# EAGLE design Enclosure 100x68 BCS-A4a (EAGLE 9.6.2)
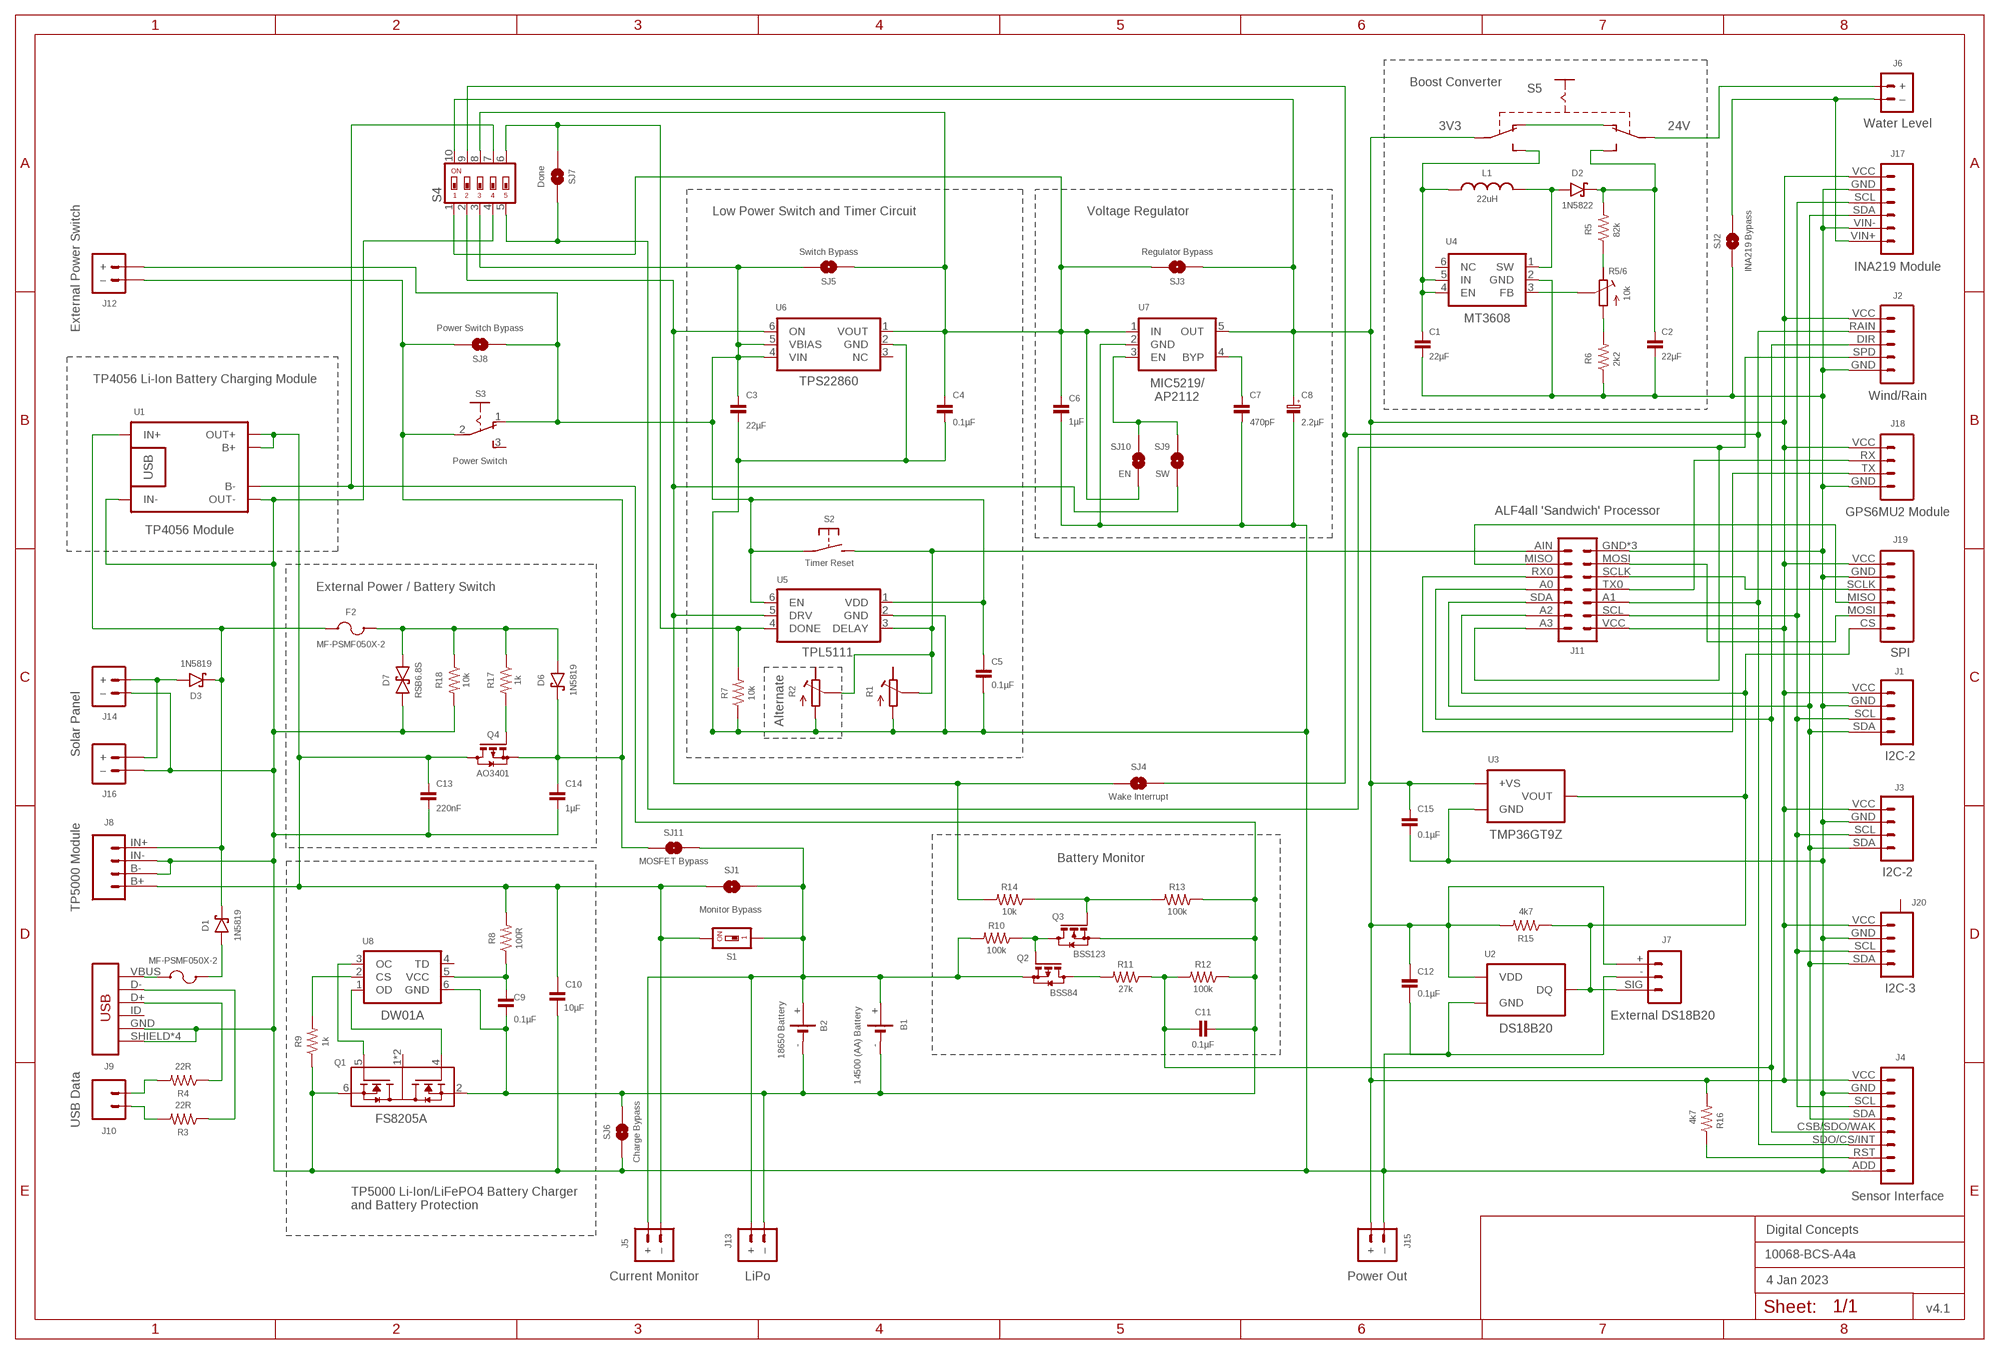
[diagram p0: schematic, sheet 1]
FRAME2 (A3L-LOC): DATE: 4 Jan 2023; OWNER: Digital Concepts; TITLE: 10068-BCS-A4a; VERSION: v4.1

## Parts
B1  14500 (AA) Battery  BATTERY-HOLDER-14500(AA)  [BATTERY-14500]
B2  18650 Battery  BATTERY-HOLDER-18650  [BATTERY-18650]
C1  22µF  CAPACITOR-1206  [C1206]
C2  22µF  CAPACITOR-1206  [C1206]
C3  22µF  CAPACITOR-0805  [C0805]
C4  0.1µF  CAPACITOR-0805  [C0805]
C5  0.1µF  CAPACITOR  [C0805@1]
C6  1µF  CAPACITOR-0805  [C0805]
C7  470pF  CAPACITOR-0805  [C0805]
C8  2.2µF  CAPACITOR-1206-TANTALUM  [C1206-POLARISED]
C9  0.1µF  CAPACITOR-0805  [C0805]
C10  10µF  CAPACITOR-VIA-2  [C0805-VIA-2@1]
C11  0.1µF  CAPACITOR-0805  [C0805]
C12  0.1µF  CAPACITOR-VIA-2  [C0805-VIA-2@1]
C13  220nF  CAPACITOR-0805  [C0805]
C14  1µF  CAPACITOR-0805  [C0805]
C15  0.1µF  CAPACITOR-0805  [C0805]
D1  1N5819  DIODE-SCHOTTKY-1N5819  [SOD-123]
D2  1N5822  DIODE-SCHOTTKY-1N5822  [DIODE_SMB]
D3  1N5819  DIODE-SCHOTTKY-1N5819  [SOD-123]
D6  1N5819  DIODE-SCHOTTKY-1N5819  [SOD-123]
D7  RSB6.8S  DIODE-SCHOTTKY-BIDIRECTIONAL  [VMD2]
F1  MF-PSMF050X-2  [F0805]
F2  MF-PSMF050X-2  [F0805]
J1  I2C-2  JST-PH2.0-4-DUAL-I2C  [JST-PH2.0-4-DUAL-I2C]
J2  Wind/Rain  JST-PH2.0-5-DUAL-WEATHER  [JST-PH2.0-5-DUAL-WEATHER]
J3  I2C-2  HEADER-1X4-I2C  [CONN_04-I2C]
J4  Sensor Interface  HEADER-1X8-SENSOR  [CONN_08-SENSOR]
J5  Current Monitor  JST-PH2.0-2-MALE-HORIZONTALJST-PTH-2  [JST-PH2.0-2-HORIZONTAL]
J6  Water Level  JST-PH2.0-2-MALE-VERTICAL  [JST-PH2.0-2-VERTICAL]
J7  External DS18B20  JST-PH2.0-DS18B20-HORIZONTAL  [JST-PH2.0-DS18B20-HORIZONTAL]
J8  TP5000 Module  HEADER-1X4-TP5000  [CONN_04-TP5000]
J9  USB  USB_MINI-B_SMT  [USB-MINIB]
J10  USB Data  1X2-PIN-HEADER  [CONN_02-GENERIC]
J11  ALF4all 'Sandwich' Processor  ALF4ALL-PROCESSOR-BOARD  [ALF4ALL-PROCESSOR-BOARD]
J12  External Power Switch  JST-PH2.0-2-DUAL-POWERJST-PTH-2  [JST-PH2.0-2-DUAL-POWER]
J13  LiPo  JST-PH2.0-2-MALE-HORIZONTALJST-PTH-2  [JST-PH2.0-2-HORIZONTAL]
J14  Solar Panel  JST-PH2.0-2-VERTICAL  [JST-PH2.0-2-VERTICAL=POWER]
J15  Power Out  JST-SH1.25-2-VERTICAL  [JST-SH1.25-2-VERTICAL]
J16  JST-PH2.0-2-HORIZONTAL-POWERJST-PTH-2  [JST-PH2.0-2-HORIZONTAL-POWER]
J17  INA219 Module  INA219-I2C-MODULE  [CONN_06-INA219]
J18  GPS6MU2 Module  HEADER-1X4-GPS  [CONN_04-GPS]
J19  SPI  JST-PH2.0-6-HORIZONTAL-SPI  [JST-PH2.0-6-HORIZONTAL-SPI]
J20  I2C-3  JST-SH1.0-4-I2C-HORIZONTAL  [JST-SH1.0-4-I2C-HORIZONTAL]
L1  22uH  INDUCTOR-CDRH104R/6D28L5038P  [CDRH104R+6D28]
Q1  FS8205A  MOSFET-DUAL-FS8205A  [FS8205-SOP?]
Q2  BSS84  [SOT23-3@1]
Q3  BSS123  MOSFET-BSS123  [SOT23-3]
Q4  AO3401  MOSFET-AO3401  [SOT-23]
R1  RESISTOR-TRIMM-BAOTER-VERTICAL  [RTRIM3296]
R2  RESISTOR-TRIMM-33  [RTRIM3*3]
R3  22R  RESISTOR-VIA-1  [R0805-VIA-1]
R4  22R  RESISTOR-VIA-1  [R0805-VIA-1]
R5  82k  RESISTORR0805  [R0805]
R5/6  10k  RESISTOR-TRIMM-BAOTER-HORIZONTAL  [RTRIM64P]
R6  2k2  RESISTORR0805  [R0805]
R7  10k  RESISTORR0805  [R0805]
R8  100R  RESISTORR0805  [R0805]
R9  1k  RESISTORR0805  [R0805]
R10  100k  RESISTORR0805  [R0805]
R11  27k  RESISTORR0805  [R0805]
R12  100k  RESISTORR0805  [R0805]
R13  100k  RESISTORR0805  [R0805]
R14  10k  RESISTORR0805  [R0805]
R15  4k7  RESISTORR0805  [R0805]
R16  4k7  RESISTORR0805  [R0805]
R17  1k  RESISTORR0805  [R0805]
R18  10k  RESISTORR0805  [R0805]
S1  Monitor Bypass  SWITCH-DIP-SWS001-VIA-1  [SMD-001-VIA-1]
S2  Timer Reset  SWITCH-MOMENTARY-2-PIN-VIA-1  [SWITCH-2-PAD-VIA-1]
S3  Power Switch  SWITCH-SLIDE-SPDT  [SWITCH-SPDT-PTH]
S4  SWITCH-DIP-SWS005  [SMD-005]
S5  SWITCH-SLIDE-DPDT-PTH-S  [SWITCH-DPDT-PTH]
SJ1  Monitor Bypass  SJ  [SJ]
SJ2  INA219 Bypass  SJ  [SJ]
SJ3  Regulator Bypass  SJ-V-12  [SJ-VIA-12]
SJ4  Wake Interrupt  SJ-V-1  [SJ-VIA-1]
SJ5  Switch Bypass  SJ-V-1  [SJ-VIA-1]
SJ6  Charge Bypass  SJ-V-1  [SJ-VIA-1]
SJ7  Done  SJ-V-1  [SJ-VIA-1]
SJ8  Power Switch Bypass  SJ  [SJ]
SJ9  SW  SJ  [SJ]
SJ10  EN  SJ  [SJ]
SJ11  MOSFET Bypass  SJ  [SJ]
U1  TP4056 Module  BATTERY-CHARGER-LI-PROT  [BATTERY-CHARGER-LI-PROT]
U2  DS18B20  THERMOMETER-DS18B20  [TO-92]
U3  TMP36GT9Z  THERMOMETER-TMP35GT9Z  [TO-92]
U4  MT3608  [SOT-23-6]
U5  TPL5111  TPL5111DDCR  [SOT-23-6]
U6  TPS22860  [SOT-23-6]
U7  MIC5219  [SOT-23-5]
U8  DW01A  [SOT-23-6]

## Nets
GND: C1.2 C2.2 C3.2 C4.1 C5.1 C6.2 C7.2 C8.2(-) C10.2 C10.2@VIA C12.2 C12.2@VIA C13.2 C14.2 C15.2 D7.P$2 J1.GND J2.GND J3.GND J4.ADD J4.GND J7.- J8.B- J8.IN- J9.GND J9.SHIELD J9.SHIELD@2(SHIELD) J9.SHIELD@3(SHIELD) J9.SHIELD@4(SHIELD) J11.GND J11.GND@TL J11.GND@TR J14.-(–) J15.-(–) J16.-(–) J17.GND J17.VIN- J18.GND J19.GND J20.GND Q1.6(S2) R1.1(A) R2.1(A) R6.1 R7.1 R9.1 R18.2 S4.4 SJ2.1 SJ6.1 SJ6.1@V U1.IN- U1.OUT- U2.1(GND) U3.3(GND) U4.2(GND) U5.2(GND) U6.2(GND) U7.2(GND)
N$1: D3.A J14.+ J16.+
N$2: C4.2 C6.1 S4.1 S4.8 SJ3.2 SJ3.2@V SJ5.1 SJ5.1@V SJ10.2 U6.1(VOUT) U7.1(IN)
N$3: R9.2 U8.2(CS)
N$4: J10.2 R4.2
N$5: R7.2 S4.6 SJ7.1 SJ7.1@V U5.4(DONE)
N$6: D2.A L1.1 U4.1(SW)
N$7: C7.1 U7.4(BYP)
N$8: J1.SCL J3.SCL J4.SCL J11.SCL J17.SCL J20.SCL
N$9: J4.RST R16.1
N$10: C11.1 J2.DIR J4.CSB/SDO/WAK J11.A0 R11.1 R12.2
N$11: J1.SDA J3.SDA J4.SDA J11.SDA J17.SDA J20.SDA
N$12: B1.+ B2.+ J5.+ J13.+ Q2.2(S) R10.2 S1.1 S1.1@VIA SJ1.1 SJ11.2
N$13: R5.1 R5/6.3(E)
N$14: J11.TX0 J18.RX
N$15: J6.-(–) J17.VIN+ SJ2.2
N$16: J11.RX0 J18.TX
N$18: Q1.5(G2) U8.3(OC)
N$19: F1.2 J9.VBUS
N$20: Q1.4(G1) U8.1(OD)
N$21: J9.D+ R4.1 R4.1@VIA
N$22: C9.1 R8.1 U8.5(VCC)
N$23: Q2.3(D) R11.2
N$24: J9.D- R3.1 R3.1@VIA
N$25: J11.AIN R1.2(S) R2.2(S) S2.2(S) U5.3(DELAY)
N$26: C3.1 C5.2 J12.+ S2.1(P) S2.1@VIA(P) S3.1(O) S4.3 SJ5.2 SJ8.1 U5.1(VDD) U5.6(EN) U6.4(VIN) U6.5(VBIAS)
N$27: R5/6.1(A) R6.2
N$28: R14.2 S4.2 SJ4.2 SJ9.2 U5.5(DRV) U6.6(ON)
N$29: J2.SPD J11.A3 S4.5 SJ7.2
N$30: J2.RAIN J4.SDO/CS/INT J11.A1 S4.9 SJ4.1 SJ4.1@V
N$31: R5/6.2(S) U4.3(FB)
N$32: C2.1 D2.C R5.2 S5.P$6(S2)
N$33: S5.P$1(O1) S5.P$4(O2)
N$34: C10.1 C13.1 J5.-(–) J8.B+ Q4.3(D) R8.2 S1.2 SJ1.2 U1.B+ U1.OUT+
N$35: Q2.1(G) Q3.3(D) R10.1
N$36: J6.+ S5.P$5(P2)
N$37: Q3.1(G) R13.2 R14.1
N$38: B1.- B2.- C9.2 C11.2 J13.-(–) Q1.2(S1) Q3.2(S) R12.1 R13.1 S4.7 SJ6.2 U1.B- U8.6(GND)
N$39: C1.1 L1.2 S5.P$3(S1) U4.4(EN) U4.5(IN)
N$40: C14.1 D6.C J12.-(–) Q4.2(S) S3.2(P) SJ8.2 SJ11.1
N$41: D1.C D3.C F2.1 J8.IN+ U1.IN+
N$42: J10.1 R3.2
N$43: Q4.1(G) R17.2
N$44: D6.A D7.P$1 F2.2 R17.1 R18.1
N$45: D1.A F1.1
N$46: SJ9.1 SJ10.1 U7.3(EN)
N$47: J11.SCLK J19.SCLK
N$48: J11.MOSI J19.MOSI
N$49: J7.SIG J11.A2 J19.CS R15.1 U2.2(DQ) U3.2(VOUT)
N$50: J11.MISO J19.MISO
VCC: C8.1(+) C12.1 C15.1 J1.VCC J2.VCC J3.VCC J4.VCC J7.+ J11.VCC J15.+ J17.VCC J18.VCC J19.VCC J20.VCC R15.2 R16.2 S4.10 S5.P$2(P1) SJ3.1 SJ3.1@V U2.3(VDD) U3.1(+VS) U7.5(OUT)
Unconnected: J9.ID J20.A@1(A) J20.A@4(A) Q1.1(D12) Q1.8(D12) R1.3(E) R2.3(E) S3.3(S) U4.6(NC) U6.3(NC) U8.4(TD)

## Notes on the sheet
- Boost Converter
- 3V3 | 24V
- Low Power Switch and Timer Circuit | Voltage Regulator
- TP4056 Li-Ion Battery Charging Module
- MIC5219/
  AP2112
- External Power / Battery Switch
- Alternate
- Battery Monitor
- TP5000 Li-Ion/LiFePO4 Battery Charger
  and Battery Protection

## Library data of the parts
B1 = digitalconcepts:BATTERY-HOLDER-14500(AA): 14500 (AA) battery holder
B2 = digitalconcepts:BATTERY-HOLDER-18650: 18650 Battery Holder
C1 C2 = digitalconcepts:CAPACITOR-1206: 1206 Capacitor
C3 C4 C6 C7 C9 C11 C13-C15 = digitalconcepts:CAPACITOR-0805: 0805 Capacitor
C5 = digitalconcepts:CAPACITOR: 0805 Capacitor
C8 = digitalconcepts:CAPACITOR-1206-TANTALUM: Capacitor 1206 Tantalum
C10 C12 = digitalconcepts:CAPACITOR-VIA-2: 0805 Capacitor with via on Pad 2
D1 D3 D6 = digitalconcepts:DIODE-SCHOTTKY-1N5819: 1N5819 Schottky Diode SOD-123
D2 = digitalconcepts:DIODE-SCHOTTKY-1N5822: 1N5822 Schottky Diode SMB
D7 = digitalconcepts:DIODE-SCHOTTKY-BIDIRECTIONAL: Schottky Bidirectional Diode
F1 F2 = digitalconcepts:MF-PSMF050X-2: PTC Resettable Fuse
J1 = digitalconcepts:JST-PH2.0-4-DUAL-I2C: PH2.0 4P I2C Dual Connector
J2 = digitalconcepts:JST-PH2.0-5-DUAL-WEATHER: PH2.0 5P Vertical Connector
J3 = digitalconcepts:HEADER-1X4-I2C: I2C Interface [Pin 1 Vcc] 4-Pin Header
J4 = digitalconcepts:HEADER-1X8-SENSOR: IoT Sensors 1x8 Pin Header for 'Sandwich' IoT Sensors
J5 J13 = digitalconcepts:JST-PH2.0-2-MALE-HORIZONTAL: PH2.0 2P Right Angle PCB Connector; PROD_ID: CONN-09863; SKU: PRT-09914
J6 = digitalconcepts:JST-PH2.0-2-MALE-VERTICAL: PH2.0 2P PCB Connector
J7 = digitalconcepts:JST-PH2.0-DS18B20-HORIZONTAL: DS18B20 PH2.0 Right Angle PCB Connector
J8 = digitalconcepts:HEADER-1X4-TP5000: TP5000 Module 4-Pin Header
J9 = digitalconcepts:USB_MINI-B: USB Mini-B Connector Breaks out 5 pins, and includes shield pins if needed.
J10 = digitalconcepts:1X2-PIN-HEADER: Single Row 2-Pin Header
J11 = digitalconcepts:ALF4ALL-PROCESSOR-BOARD: ALF4all 'Sandwixh' Processor 2x7 Pin Header and earthed 1x1 locator pins for ALF4all 'Sandwich' Processor/RFM95W PCBs
J12 = digitalconcepts:JST-PH2.0-2-DUAL-POWER: JST PH2.0 2P PTH Dual-Side Connector (Power); PROD_ID: CONN-09863; SKU: PRT-09914
J14 = digitalconcepts:JST-PH2.0-2-VERTICAL: PH2.0 2P PCB Connector
J15 = digitalconcepts:JST-SH1.25-2-VERTICAL: SH1.25 Male PCB Connector
J16 = digitalconcepts:JST-PH2.0-2-HORIZONTAL-POWER: PH2.0 2P Right Angle PCB Connector; PROD_ID: CONN-09863; SKU: PRT-09914
J17 = digitalconcepts:INA219-I2C-MODULE: INA219 I2C Module
J18 = digitalconcepts:HEADER-1X4-GPS: NEO GPS 4-Pin Header
J19 = digitalconcepts:JST-PH2.0-6-HORIZONTAL-SPI: PH2.0 6P Horizontal Connector—SPI
J20 = digitalconcepts:JST-SH1.0-4-I2C-HORIZONTAL: JST SH1.0 SMD 4P I2C horizontal connector
L1 = digitalconcepts:INDUCTOR-CDRH104R/6D28: Inductor; SPICEPREFIX: L
Q1 = digitalconcepts:MOSFET-DUAL-FS8205A: Dual MOSFET; AVAILABILITY: Unavailable; MF: Fortune Semiconductor; MP: FS8205A; PACKAGE: Package; PRICE: None
Q2 = digitalconcepts:BSS84: P-CHANNEL MOS FET
Q3 = digitalconcepts:MOSFET-BSS123: N-CHANNEL MOS FET
Q4 = digitalconcepts:MOSFET-AO3401: AO3401 P-Channel MOSFET
R1 = digitalconcepts:RESISTOR-TRIMM-BAOTER-VERTICAL: Trimm Resistor - Vertical BAOTER
R2 = digitalconcepts:RESISTOR-TRIMM-3*3: Trimm Resistor - 3*3 SMD
R3 R4 = digitalconcepts:RESISTOR-VIA-1: Resistor with via on Pad 1
R5-R18 = digitalconcepts:RESISTOR: Resistor; SPICEPREFIX: R
R5/6 = digitalconcepts:RESISTOR-TRIMM-BAOTER-HORIZONTAL: Trimm Resistor - Horizontal BAOTER
S1 = digitalconcepts:SWITCH-DIP-SWS001-VIA-1: SMD Dip Switch 1 pol.
S2 = digitalconcepts:SWITCH-MOMENTARY-2-PIN-VIA-1: 2 Pin Momentary Switch
S3 = digitalconcepts:SWITCH-SLIDE-SPDT: Mini Sliding Switch SPDT
S4 = digitalconcepts:SWITCH-DIP-SWS005: SMD Dip Switch 5 pol.
S5 = digitalconcepts:SWITCH-SLIDE-DPDT-PTH-S: Switch DPDT PTH-S
SJ1 SJ2 SJ8-SJ11 = digitalconcepts:SJ: Solder Jumper
SJ3 = digitalconcepts:SJ-V-12: Solder Jumper with Pad Vias
SJ4-SJ7 = digitalconcepts:SJ-V-1: Solder Jumper with single Pad Via
U1 = digitalconcepts:BATTERY-CHARGER-LI-PROT: TP4056 Li Battery Charger module with PCB (rather than module) footprint
U2 = digitalconcepts:THERMOMETER-DS18B20: Digital Thermometer -55C-125C TO92-3; AVAILABILITY: Bad; DESCRIPTION: Temperature Sensor Digital, Local -55°C ~ 125°C 12 b 8-uMAX; MF: Maxim Integrated; MP: DS18B20; PACKAGE: TO-92 Maxim Integrated; PRICE: None
U3 = digitalconcepts:THERMOMETER-TMP35GT9Z: Temperature Sensor; AVAILABILITY: Warning; DESCRIPTION: Temperature Sensor Analog, Local 10°C ~ 125°C 10mV/°C TO-92-3; MF: Analog Devices; MOUSER-PURCHASE-URL: https://snapeda.com/shop?store=Mouser&id=409845; MP: TMP35GT9Z; PACKAGE: TO-92-3 Analog Devices; PRICE: None
U4 = digitalconcepts:MT3608: MT3608 DC-DC Step-Up Voltage Converter
U5 = digitalconcepts:TPL5111DDCR: TPL5111 Nano-Power System Timer
U6 = digitalconcepts:TPS22860: Texas Instruments TPS22860 Ultra-Low Leakage Load Switch
U7 = digitalconcepts:MIC5219: Microchip LDO Linear Voltage Regulator; OC_FARNELL: unknown; OC_NEWARK: unknown
U8 = digitalconcepts:DW01A: Battery Protection IC; AVAILABILITY: Unavailable; DESCRIPTION: One Cell Lithium-ion/Polymer Battery Protection IC; MF: Fortune Semiconductor; MP: DW01A; PACKAGE: SOT-23-6 Fortune Semiconductor; PRICE: None

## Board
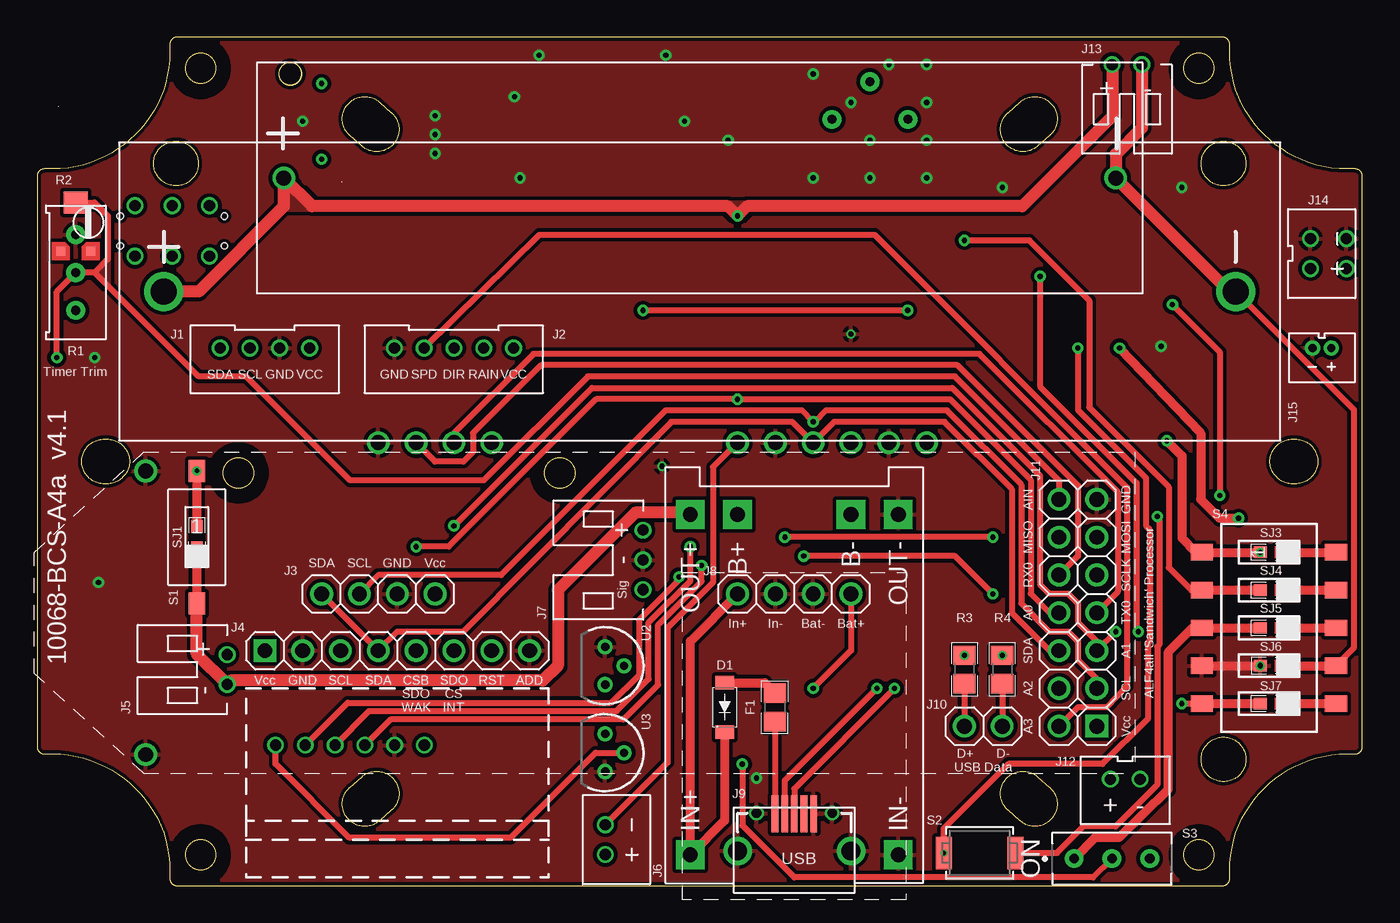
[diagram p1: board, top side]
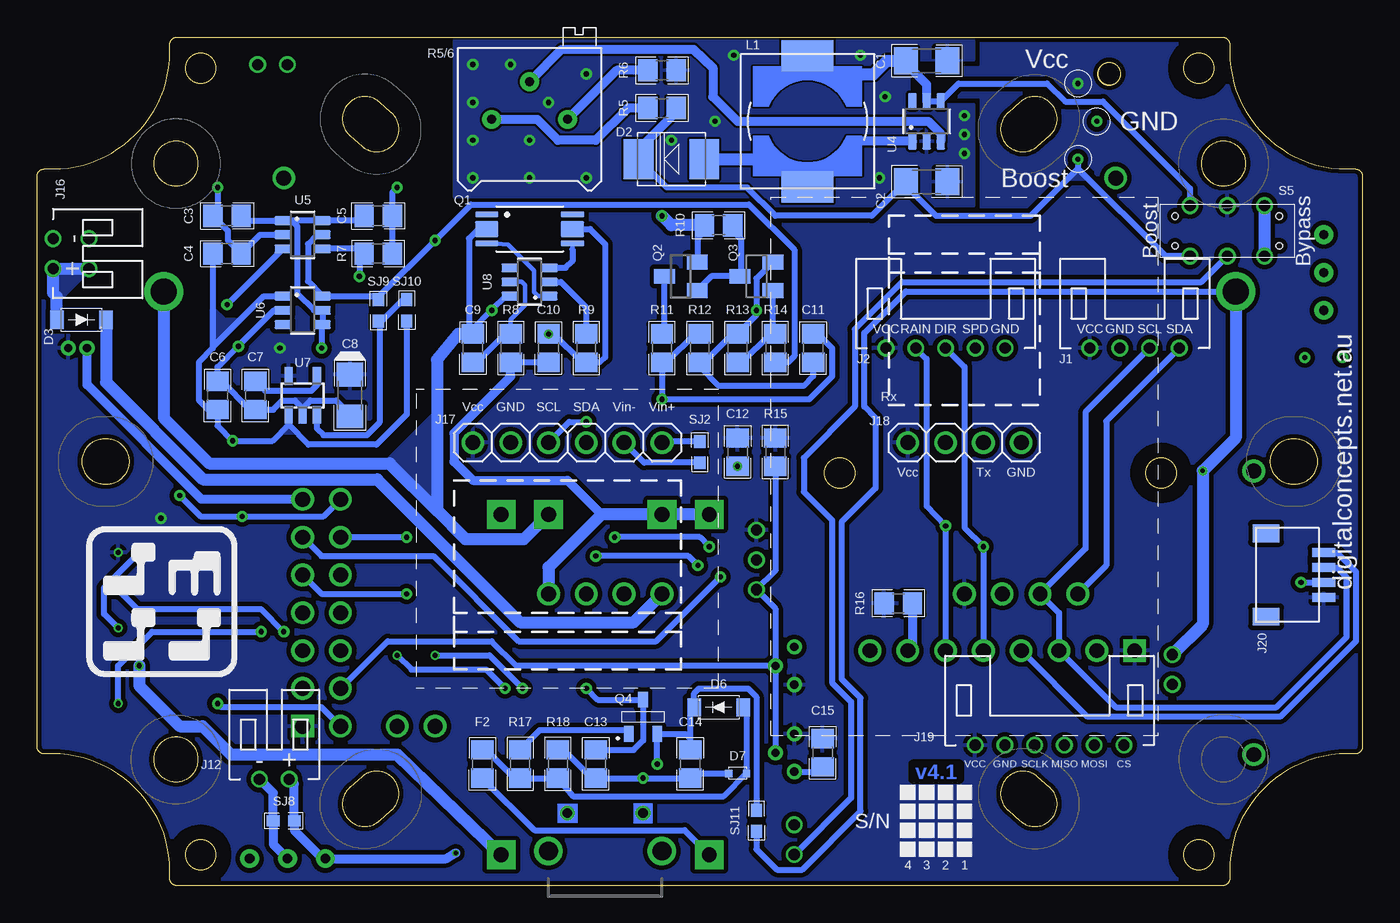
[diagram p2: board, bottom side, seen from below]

Size 89 x 57 mm. Coordinates in mm from the lower left corner, seen from the top.
Outline: 1146 segments
Outline: circle at 17,54.54 radius 0.76
Outline: circle at 10.97,54.91 radius 1.02
Outline: circle at 10.97,2.08 radius 1.02
Outline: circle at 13.51,27.73 radius 1.02
Outline: circle at 35.1,27.73 radius 1.02
Outline: circle at 78.03,2.08 radius 1.02
Outline: circle at 78.03,54.91 radius 1.02
Copper layers (1*16): Top 0.035mm / dielectric 1.5mm / Bottom 0.035mm
Design rules "default *": minimum track width 6mil, minimum drill 0.3mm, track to track 6mil, track to pad 6mil, pad to pad 6mil, via to via 6mil, smd to smd 6mil, copper to edge 6mil, drill to drill 6mil, minimum pad ring 1mil, minimum via ring 8mil, stop-mask expansion 4mil, vias tented up to drill 0mil, thermal gap 10mil

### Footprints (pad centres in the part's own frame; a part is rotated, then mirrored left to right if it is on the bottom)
BATTERY-14500 = drill 1: + -27.94,0; - 27.94,0
BATTERY-18650 = drill 1.75: + -36,0; - 36,0
C1206 = smd 1.6 x 1.8: 1 -1.4,0; 2 1.4,0
C0805 = smd 1.3 x 1.5: 1 -0.95,0; 2 0.95,0
C0805@1 = smd 1.3 x 1.5: 1 -0.95,0; 2 0.95,0
C1206-POLARISED = smd 1.6 x 1.8: 1 -1.4,0; 2 1.4,0
C0805-VIA-2@1 = smd 1.3 x 1.5: 1 -0.95,0; 2 0.95,0 | drill 0.35 pad 0.61: 2@VIA 0.95,0
SOD-123 = smd 0.91 x 1.22: A -1.65,0; C 1.65,0
DIODE_SMB = smd 2 x 2.7: A 2.2,0; C -2.2,0
VMD2 = smd 0.5 x 0.5: P$1 -0.6,0; P$2 0.6,0
F0805 = smd 1.3 x 1.5: 1 -0.95,0; 2 0.95,0
JST-PH2.0-4-DUAL-I2C = drill 0.75: GND -1,0; SCL 1,0; SDA 3,0; VCC -3,0
JST-PH2.0-5-DUAL-WEATHER = drill 0.75: DIR 0,0; GND 4,0; RAIN -2,0; SPD 2,0; VCC -4,0
CONN_04-I2C = drill 1 pad 1.524: GND 2.54,0; SCL 5.08,0; SDA 7.62,0; VCC 0,0
CONN_08-SENSOR = drill 1 pad 1.524: ADD 17.78,0; CSB/SDO/WAK 10.16,0; GND 2.54,0; RST 15.24,0; SCL 5.08,0; SDA 7.62,0; SDO/CS/INT 12.7,0 | drill 1 pad 1.524 square: VCC 0,0
JST-PH2.0-2-HORIZONTAL = drill 0.75: + 1,0; - -1,0
JST-PH2.0-2-VERTICAL = drill 0.75: + -1,0; - 1,0
JST-PH2.0-DS18B20-HORIZONTAL = drill 0.75: + 2,0; - 0,0; SIG -2,0
CONN_04-TP5000 = drill 1 pad 1.524: B+ 0,0; B- 2.54,0; IN+ 7.62,0; IN- 5.08,0
USB-MINIB = smd 2.5 x 0.45: D+ 2.5,0; D- 2.5,0.65; GND 2.5,-1.3; ID 2.5,-0.65; VBUS 2.5,1.3 | drill 1.27: SHIELD 0,3.81; SHIELD@2 0,-3.81 | drill 0.65 pad 0.762: SHIELD@3 2.54,2.54; SHIELD@4 2.54,-2.54
CONN_02-GENERIC = drill 1 pad 1.524: 1 0,0; 2 2.54,0
ALF4ALL-PROCESSOR-BOARD = drill 1 pad 1.524: A0 7.62,2.54; A1 5.08,0; A2 2.54,2.54; A3 0,2.54; AIN 15.24,2.54; GND 15.24,0; GND@TL -1.905,63.881; GND@TR 17.145,63.881; MISO 12.7,2.54; MOSI 12.7,0; RX0 10.16,2.54; SCL 2.54,0; SCLK 10.16,0; SDA 5.08,2.54; TX0 7.62,0 | drill 1 pad 1.524 square: VCC 0,0
JST-PH2.0-2-DUAL-POWER = drill 0.75: + 1,0; - -1,0
JST-PH2.0-2-VERTICAL=POWER = drill 0.75: + -1,0; - 1,0
JST-SH1.25-2-VERTICAL = drill 0.55 pad 1.016: + 0.625,0; - -0.625,0
JST-PH2.0-2-HORIZONTAL-POWER = drill 0.75: + 1,0; - -1,0
CONN_06-INA219 = drill 1 pad 1.524: GND 2.54,0; SCL 5.08,0; SDA 7.62,0; VCC 0,0; VIN+ 12.7,0; VIN- 10.16,0
CONN_04-GPS = drill 1 pad 1.524: GND 0,0; RX 5.08,0; TX 2.54,0; VCC 7.62,0
JST-PH2.0-6-HORIZONTAL-SPI = drill 0.75: CS 5,0; GND -3,0; MISO 1,0; MOSI 3,0; SCLK -1,0; VCC -5,0
JST-SH1.0-4-I2C-HORIZONTAL = smd 1.2 x 1.8: A@1 -2.8,-3.875; A@4 2.8,-3.875 | smd 0.6 x 1.55: GND 0.5,0; SCL -0.5,0; SDA -1.5,0; VCC 1.5,0
CDRH104R+6D28 = smd 2.1 x 3.5: 1 -4.4,0; 2 4.4,0
FS8205-SOP? = smd 1.56 x 0.4: 1 -2.88,0.975; 4 -2.88,-0.975; 5 2.88,-0.975; 8 2.88,0.975 | smd 1.56 x 1.05: 2 -2.88,0; 6 2.88,0
SOT23-3@1 = smd 1 x 1.4: 1 -0.95,-1.1; 2 0.95,-1.1; 3 0,1.1
SOT23-3 = smd 1 x 1.4: 1 -0.95,-1.1; 2 0.95,-1.1; 3 0,1.1
SOT-23 = smd 0.65 x 1.05: 1 -0.95,-1.15; 2 0.95,-1.15; 3 0,1.15
RTRIM3296 = drill 0.61 pad 1.27: 1 0,-2.54; 2 0,0; 3 0,2.54
RTRIM3*3 = smd 0.6 x 0.6: 1 -1,-1.6; 3 1,-1.6 | smd 1.6 x 1.5: 2 0,1.65
R0805-VIA-1 = smd 1.3 x 1.5: 1 -0.95,0; 2 0.95,0 | drill 0.35 pad 0.61: 1@VIA -0.95,0
R0805 = smd 1.3 x 1.5: 1 -0.95,0; 2 0.95,0
RTRIM64P = drill 0.61 pad 1.27: 1 0,-2.54; 2 2.54,0; 3 0,2.54
SMD-001-VIA-1 = smd 1.1 x 1.5: 1 0,-4.45; 2 0,4.45 | drill 0.3 pad 0.61: 1@VIA 0,-4.45
SWITCH-2-PAD-VIA-1 = smd 1.067 x 2.184: 1 -2.4,0; 2 2.4,0 | drill 0.3: 1@VIA -2.4,0
SWITCH-SPDT-PTH = drill 0.65 pad 1.27: 1 -2.54,0; 2 0,0; 3 2.54,0
SMD-005 = smd 1.1 x 1.5: 1 -5.08,-4.5; 2 -2.54,-4.5; 3 0,-4.5; 4 2.54,-4.5; 5 5.08,-4.5; 6 5.08,4.5; 7 2.54,4.5; 8 0,4.5; 9 -2.54,4.5; 10 -5.08,4.5
SWITCH-DPDT-PTH = drill 0.75: P$1 -1.7,2.5; P$2 -1.7,0; P$3 -1.7,-2.5; P$4 1.7,2.5; P$5 1.7,0; P$6 1.7,-2.5 | hole 0.42: 1,3.5; -1,3.5; 1,-3.5; -1,-3.5
SJ = smd 0.864 x 0.762: 1 -0.711,0; 2 0.711,0
SJ-VIA-12 = smd 0.864 x 0.762: 1 -0.711,0; 2 0.711,0 | drill 0.35 pad 0.61: 1@V -0.711,0; 2@V 0.711,0
SJ-VIA-1 = smd 0.864 x 0.762: 1 -0.711,0; 2 0.711,0 | drill 0.35 pad 0.61: 1@V -0.711,0
BATTERY-CHARGER-LI-PROT = drill 1 pad 1.93 square: B+ 10.795,3.81; B- 10.795,-3.81; IN+ -12.065,6.985; IN- -12.065,-6.985; OUT+ 10.795,6.985; OUT- 10.795,-6.985
TO-92 = drill 0.55 pad 1.016: 1 -1.27,0; 2 0,1.27; 3 1.27,0
SOT-23-6 = smd 1.1 x 0.6: 1 -1.35,0.95; 2 -1.35,0; 3 -1.35,-0.95; 4 1.35,-0.95; 5 1.35,0; 6 1.35,0.95
SOT-23-5 = smd 0.55 x 1.2: 1 -0.95,-1.3; 2 0,-1.3; 3 0.95,-1.3; 4 0.95,1.3; 5 -0.95,1.3

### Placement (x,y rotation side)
B1  44.5,47.54 0 top
B2  44.5,39.92 0 top
C1  29.26,55.42 0 bottom
C2  29.26,47.29 0 bottom
C3  76.25,45 180 bottom
C4  76.25,42.46 180 bottom
C5  66.09,45 180 bottom
C6  76.88,32.94 90 bottom
C7  74.34,32.94 270 bottom
C8  67.99,32.94 270 bottom
C9  59.74,36.11 90 bottom
C10  54.66,36.11 90 bottom
C11  36.88,36.11 270 bottom
C12  41.96,29.13 270 bottom
C13  51.48,8.17 270 bottom
C14  45.13,8.17 270 bottom
C15  36.24,8.93 270 bottom
D1  46.18,11.98 270 top
D2  46.4,48.81 0 bottom
D3  86.03,38.02 0 bottom
D6  43.23,11.98 180 bottom
D7  41.96,7.54 180 bottom
F1  49.55,11.98 270 top
F2  59.1,8.17 90 bottom
J1  15.29,36.11 0 bottom
J2  27.99,36.11 0 bottom
J3  26.72,19.6 180 top
J4  15.29,15.79 0 top
J5  12.75,14.52 90 top
J6  38.15,3.09 90 top
J7  40.69,21.89 90 top
J8  54.66,19.6 180 top
J9  50.85,2.33 90 top
J10  62.28,10.71 0 top
J11  71.17,10.71 90 top
J12  73.07,7.16 0 bottom
J13  73.2,55.16 180 top
J14  85.52,42.46 90 top
J15  86.28,36.11 0 top
J16  87.93,42.46 270 bottom
J17  59.74,29.76 0 bottom
J18  22.91,29.76 180 bottom
J19  21,9.44 0 bottom
J20  2.59,20.87 270 bottom
L1  37.26,51.35 90 bottom
Q1  55.93,44.11 0 bottom
Q2  45.77,40.94 90 bottom
Q3  40.69,40.94 90 bottom
Q4  48.31,11.35 0 bottom
R1  2.59,41.19 180 top
R2  2.59,44.24 0 top
R3  62.28,14.52 270 top
R4  64.82,14.52 270 top
R5  47.04,52.24 0 bottom
R5/6  55.93,51.48 90 bottom
R6  47.04,54.78 180 bottom
R7  66.09,42.46 180 bottom
R8  57.2,36.11 270 bottom
R9  52.12,36.11 90 bottom
R10  43.23,44.37 180 bottom
R11  47.04,36.11 90 bottom
R12  44.5,36.11 90 bottom
R13  41.96,36.11 270 bottom
R14  39.42,36.11 270 bottom
R15  39.42,29.13 90 bottom
R16  31.16,18.97 180 bottom
R17  56.56,8.17 90 bottom
R18  54.02,8.17 90 bottom
S1  10.72,23.41 180 top
S2  63.3,2.2 0 top
S3  72.19,1.82 0 top
S4  82.73,17.32 270 top
S5  9.07,43.99 270 bottom
SJ1  10.72,23.41 270 top
SJ2  44.5,29.13 90 bottom
SJ3  82.85,22.4 180 top
SJ4  82.85,19.86 180 top
SJ5  82.85,17.32 180 top
SJ6  82.85,14.78 0 top
SJ7  82.85,12.24 180 top
SJ8  72.44,4.36 180 bottom
SJ9  66.09,38.65 90 bottom
SJ10  64.18,38.65 270 bottom
SJ11  40.69,4.36 270 bottom
U1  50.85,14.14 90 top
U2  38.15,14.78 270 top
U3  38.15,8.93 270 top
U4  29.26,51.35 90 bottom
U5  71.17,43.73 0 bottom
U6  71.17,38.65 0 bottom
U7  71.17,32.94 0 bottom
U8  55.93,40.56 180 bottom

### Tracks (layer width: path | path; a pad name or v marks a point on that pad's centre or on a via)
$X0
  cutout Bottom: 10.97,56.94 arc180 10.97,52.88 arc180
$X1
  cutout Bottom: 78.03,56.94 arc180 78.03,52.88 arc180
$X2
  cutout Bottom: 78.03,4.11 arc180 78.03,0.04 arc180
$X3
  cutout Bottom: 10.97,4.11 arc180 10.97,0.04 arc180
$X4
  cutout Top: 10.97,56.94 arc180 10.97,52.88 arc180
$X5
  cutout Top: 78.03,56.94 arc180 78.03,52.88 arc180
$X6
  cutout Top: 78.03,4.11 arc180 78.03,0.04 arc180
$X7
  cutout Top: 10.97,4.11 arc180 10.97,0.04 arc180
$X8
  cutout Bottom: 13.51,29.76 arc180 13.51,25.7 arc180
$X9
  cutout Top: 35.1,29.76 arc180 35.1,25.7 arc180
$X10
  cutout Top: 13.51,29.76 arc180 13.51,25.7 arc180
$X11
  cutout Bottom: 35.1,29.76 arc180 35.1,25.7 arc180
GND  (via drill 0.35)
  Top 0.61: S4.4 SJ6.1@V
  Bottom 0.406: D7.P$2 44.82,7.54 C14.2 v48.31,7.22 C13.2 51.74,7.22 53.64,9.12 R18.2 | C10.2@VIA 54.3,37.06 52.4,35.16 R9.1 51.24,35.16 50.85,35.5 50.85,43.1 51.87,44.11 Q1.6 | R7.1 C5.1 65.14,46.59 v64.82,46.91 | U5.2 74.03,43.73 C4.1 76.19,43.36 76.19,43.99 C3.2 76.88,45.32 v76.88,46.91 | U3.3 36.56,7.66 C15.2 | v4.11,20.37 J20.GND | C8.2 67.99,31.67 68.92,32.59 70.64,32.59 71.17,32.07 | U6.2 73.07,38.65 v75.49,36.24 76.88,34.84 C6.2 76.63,33.89 74.73,31.99 C7.2 73.15,31.99 72.54,32.59 71.7,32.59 71.17,32.07 | U7.2 71.17,32.07 | SJ2.1 48.23,28.42 J17.VIN-
  Bottom 0.61: J15.- 85.66,33.66 77.95,25.95 J11.GND
  Bottom 0.813: U1.IN- 64.82,8.81 76,8.81 77.9,10.71 79.42,10.71 82.14,13.43 SJ6.1@V
  other vias: 26.72,51.73 26.72,50.46 26.72,49.19 46.4,50.08 32.05,53 52.12,47.54 55.93,47.54 59.74,55.16 59.74,52.62 52.12,54.53 55.93,50.08 59.74,47.54 59.74,50.08 42.21,55.8 43.48,51.35 32.43,47.54 17.83,51.35 3.86,35.48 33.7,55.8 57.2,55.16 54.66,52.62
  pour Top (isolate 0.254, rank 5): -2.92,59.5 -2.92,-2.56 91.86,-2.56 91.86,59.5
  pour Bottom (rank 2): 61.01,57.07 26.08,57.07 26.08,55.44 30.4,55.44 30.4,52.5 26.08,52.5 26.08,45.64 39.42,45.64 40.05,46.27 61.01,46.27
  pour Bottom (no thermals): 71.17,32.07 70.64,32.59 71.7,32.59
N$1
  Bottom 0.813: D3.A 87.68,39.56 87.93,39.81 J16.+ J14.+
  pour Bottom (no thermals): 87.68,41.46 85.77,41.46 87.68,39.56
N$2  (via drill 0.35)
  Top 0.61: v75.87,29.89 76.88,28.87 76.88,23.35 77.83,22.4 S4.1 SJ3.2@V | SJ5.1@V S4.8
  Bottom 0.406: 72.12,30.97 73.2,29.89 v75.87,29.89 76.88,30.91 C6.1 77.52,31.99 78.15,32.62 78.15,35.16 77.2,36.11 77.2,36.18 | SJ3.2@V 84.5,20.03 84.5,18.26 SJ5.1@V | C4.2 77.2,36.18 | 72.12,30.97 70.79,29.64 66.22,29.64 64.18,31.67 SJ10.2 | 72.12,30.97 U7.1 | 77.2,36.18 73.78,39.6 U6.1
  pour Bottom (no thermals): 77.2,38.72 76.46,37.97 75.4,37.97 77.2,36.18
  pour Bottom (no thermals): 72.56,30.52 71.68,30.52 72.12,30.97
N$3
  Bottom 0.406: U8.2 53.82,40.56 52.14,38.88 52.14,37.09 R9.2
N$4
  Top 0.406: R4.2 J10.2
N$5  (via drill 0.35)
  Top 0.406: v73.96,17.06 73.84,17.19 73.84,27.07 67.36,33.55 v67.36,40.94
  Top 0.61: SJ7.1@V S4.6
  Bottom 0.406: U5.4 66.72,42.78 R7.2 67.36,42.14 v67.36,40.94 | SJ7.1@V 83.56,14.78 81.28,17.06 v73.96,17.06
N$6
  Bottom 0.61: L1.1 36.31,48.3 35.66,48.3 33.96,50 U4.1
  Bottom 0.813: D2.A 39.9,48.81 39.42,48.3 38.21,48.3 L1.1
N$7
  Bottom 0.406: U7.4 70.22,33.6 70.57,33.25 73.71,33.25 C7.1
N$8  (via drill 0.35)
  Top 0.406: J11.SCL 71.17,13.89 69.9,15.16 69.9,16.43 69.26,17.06 67.99,17.06 66.09,18.97 66.09,26.94 61.11,31.92 52.99,31.92 52.23,31.16 v52.12,31.16 51.36,31.92 42.21,31.92 31.16,20.87 22.91,20.87 J3.SCL
  Bottom 0.406: v52.12,31.16 53.26,31.16 J17.SCL | J1.SCL 18.59,31.81 18.59,22.65 J3.SCL 20.37,18.33 J4.SCL 16.56,11.98 5.76,11.98 1.07,16.68 1.07,20.74 1.7,21.37 J20.SCL
N$9
  Bottom 0.61: J4.RST 30.21,16.11 R16.1
N$10  (via drill 0.35)
  Top 0.406: v25.45,22.78 27.63,22.78 37.54,32.68 v47.04,32.68 61.29,32.68 66.72,27.25 66.72,19.6 67.99,18.33 J11.A0
  Bottom 0.406: J4.CSB/SDO/WAK v25.45,22.78 26.72,24.05 26.72,34.84 J2.DIR | R12.2 44.83,37.06 46.73,35.16 R11.1 v47.04,32.68 37.13,32.68 35.61,34.21 35.61,36.11 36.24,36.75 36.56,36.75 C11.1
N$11
  Top 0.406: J11.SDA 67.99,15.79 65.45,18.33 65.45,26.64 60.93,31.16 53.52,31.16 J17.SDA 50.72,31.16 42.59,31.16 28.6,17.06 24.18,17.06 J4.SDA J3.SDA
  Bottom 0.406: J4.SDA 18.46,11.35 5.51,11.35 0.43,16.43 0.43,21.1 1.7,22.37 J20.SDA | J3.SDA 17.19,21.51 17.19,31.21 J1.SDA
N$12  (via drill 0.35)
  Top 0.61: S1.1@VIA SJ1.1
  Top 0.813: J13.+ 72.2,51.68 66.16,45.64 47.67,45.64 v47.04,45 46.4,45.64 18.46,45.64 B1.+ 16.56,45.64 10.84,39.92 B2.+
  Bottom 0.406: R10.2 44.18,43.96 44.64,43.5 44.64,41.92 Q2.2 | SJ11.2 40.69,2.46 39.32,1.09 37.62,1.09 33.7,5 33.7,12.62 34.97,13.89 34.97,24.43 32.69,26.71 32.69,31.41 33.45,32.18 33.45,37.13 30.66,39.92 B2.+
  Bottom 0.813: J5.+ 10.72,17.55 S1.1@VIA 8.5,30.08 B2.+ | v47.04,45 46.4,44.37 R10.2
  pour Top: 16.56,47.54 18.46,45.64 16.56,45.64
  pour Top (no thermals): 47.04,45 46.4,45.64 47.67,45.64
N$13
  Bottom 0.61: R5.1 49.33,52.24 51.48,50.08 54.02,50.08 55.42,51.48 R5/6.3
N$14
  Top 0.406: J11.TX0 72.57,19.73 72.57,26.46 63.3,35.73 33.32,35.73 27.99,30.4 J18.RX
N$15
  Top 0.406: J6.- 42.34,8.28 42.34,17.32 45.39,20.36 45.39,28.11 J17.VIN+
  Bottom 0.406: SJ2.2 46.96,29.84 J17.VIN+
N$16
  Top 0.406: J11.RX0 69.9,22.14 69.9,26.89 61.82,34.97 33.83,34.97 29.26,30.4 29.26,29.13 28.62,28.49 26.72,28.49 J18.TX
N$18
  Bottom 0.305: Q1.5 53.06,42.76
  Bottom 0.406: 53.06,42.76 53.06,41.95 53.5,41.51 U8.3
N$19
  Top 0.406: F1.2 J9.VBUS
N$20
  Bottom 0.305: U8.1 55.37,39.61 55.62,39.86 55.62,41.31 57.38,43.07 58.17,43.14 Q1.4
N$21  (via drill 0.35)
  Top 0.406: v57.58,13.25 50.85,6.52 J9.D+
  Bottom 0.406: v57.58,13.25 58.85,14.52 63.87,14.52 R4.1@VIA
N$22
  Bottom 0.305: U8.5 57.19,40.59 56.48,40.59 56.22,40.33 56.22,39.01 57.2,38.03 R8.1
  Bottom 0.406: C9.1 59.46,35.16 57.56,37.06 R8.1
N$23
  Bottom 0.406: Q2.3 46.89,40.54 46.89,37.21 R11.2
N$24  (via drill 0.35)
  Top 0.406: v56.4,13.25 50.2,7.05 J9.D-
  Bottom 0.406: R3.1@VIA 58.62,15.47 v56.4,13.25
N$25  (via drill 0.35)
  Top 0.406: 3.86,41.19 10.84,34.21 14.02,34.21 21,27.22 30,27.22 36.98,34.21 61.64,34.21 68.63,27.22 J11.AIN | v76.25,39.03 79.42,35.86 v79.42,26.21 | v75.23,24.81 75.36,24.68 75.36,16.17 75.23,16.05 75.23,6.78 72.44,3.98 70.28,3.98 68.5,2.2 S2.2 | 3.86,41.19 4.75,42.08 4.75,45 3.86,45.89 R2.2 | 3.86,41.19 R1.2 1.32,39.92 v1.32,35.48
  Bottom 0.406: v79.42,26.21 78.03,24.81 v75.23,24.81 69.77,24.81 J11.AIN | U5.3 72.52,42.76 v76.25,39.03
  pour Top: 3.86,41.19 4.75,42.08 4.75,40.3
N$26  (via drill 0.35)
  Top 0.406: S2.1@VIA 60.9,3.85 65.21,8.17 71.55,8.17 74.6,11.22 74.6,16.3 74.73,16.43 74.73,23.92 74.47,24.17 74.47,27.37 69.9,31.95 v69.9,36.11
  Top 0.61: S3.1 71.04,3.22 72.64,3.22 75.94,6.45 75.94,15.67 77.59,17.32 S4.3 SJ5.2
  Bottom 0.406: U5.1 U5.6 66.84,44.68 C5.2 | U5.1 71.91,44.68 71.53,44.3 71.53,39.77 70.41,38.65 U6.5 U6.4 69.9,37.62 v69.9,36.11 | C3.1 74.98,44.68 U5.1
  Bottom 0.61: S2.1@VIA 61.53,1.82 S3.1 69.82,1.82 71.73,3.73 SJ8.1 71.73,6.81 J12.+
N$27
  Bottom 0.61: R5/6.1 50.09,54.78 R6.2
N$28  (via drill 0.35)
  Top 0.406: v62.28,43.35 66.65,43.35 70.66,39.32 70.66,32.12 76,26.79 76,21.38 77.51,19.86 S4.2
  Top 0.61: S4.2 SJ4.2
  Bottom 0.406: U5.5 70.2,43.73 70.82,43.12 70.82,40.6 U6.6 66.33,39.6 SJ9.2 66.09,39.54 v62.28,43.35 59.87,45.76 41.2,45.76 38.15,42.72 38.15,35.57 38.56,35.16 R14.2
N$29  (via drill 0.35)
  Top 0.406: J11.A3 69.9,11.98 71.83,11.98 73.2,13.39 73.2,26.77 56.23,43.73 33.73,43.73 J2.SPD | v76.88,12.24 S4.5
  Top 0.61: S4.5 SJ7.2
  Bottom 0.406: J11.A3 69.9,11.98 76.63,11.98 v76.88,12.24
N$30  (via drill 0.35)
  Top 0.406: v72.44,17.06 J11.A1 71.17,16.43 69.9,17.7 69.9,18.97 69.26,19.6 67.99,19.6 67.36,20.24 67.36,27.55 61.47,33.45 37.26,33.45 v27.99,24.17
  Top 0.61: SJ4.1@V S4.9
  Bottom 0.406: J4.SDO/CS/INT v27.99,24.17 29.26,25.5 29.26,35.38 J2.RAIN | v72.44,17.06 73.96,18.59 82.29,18.59 SJ4.1@V
N$31
  Bottom 0.61: R5/6.2 53.77,56.18 44.91,56.18 43.61,54.96 43.61,53 41.96,51.35 29.16,51.35 28.31,50.51 U4.3
N$32  (via drill 0.35)
  Bottom 0.406: 19.1,48.18 22.27,45 28.62,45 30.66,47.04 C2.1 32.95,45 39.42,45 41.32,46.91 46.7,46.91 D2.C | S5.P$6 13.21,42.29 19.1,48.18 | v19.1,48.81 19.1,48.18
  Bottom 0.61: R5.2 46.09,51.97 48.6,49.45 D2.C
  pour Bottom (no thermals): 19.1,48.18 18.46,47.54 19.73,47.54
N$33
  Bottom 0.813: S5.P$1 S5.P$4
N$34  (via drill 0.35)
  Top 0.406: J8.B+ 54.66,15.79 v52.12,13.25
  Top 0.61: SJ1.2 S1.2
  Top 0.813: S1.2 10.72,15.55 J5.- 13,13.78 33.97,13.78 34.97,14.78 34.97,19.86 40.18,25.06 43.74,25.06 U1.OUT+
  Bottom 0.406: C13.1 48.94,9.12 48.31,9.76 Q4.3 51.36,12.5 v52.12,13.25 | R8.2 C10.1
  Bottom 0.61: R8.2 57.2,34.21 61.01,30.4 61.01,28.49 59.74,27.22 53.39,27.22 51.1,24.94
  Bottom 0.813: J8.B+ 54.66,21.38 51.1,24.94 U1.B+ U1.OUT+
N$35
  Bottom 0.406: R10.1 42.28,43.99 41.71,43.42 41.71,41.01 Q3.3 43.72,40.94 Q2.1
N$36
  Bottom 0.406: J6.+ 34.34,5.9 34.34,12.36 35.61,13.63 35.61,24.56 37.51,26.46 37.51,28.75 34.09,32.18 34.09,37.38 30.91,40.56 10.8,40.56 S5.P$5
N$37
  Bottom 0.406: R13.2 41.93,35.13 41.68,35.13 39.75,37.06 R14.1 39.62,37.27 39.62,39.96 Q3.1
N$38  (via drill 0.35)
  Top 0.406: B2.- 88.44,31.98 88.44,15.99 S4.7 | v40.69,38.65 v58.47,38.65
  Top 0.61: SJ6.2 S4.7
  Top 0.813: J13.- 74.2,50.92 72.44,49.16 B1.- 80.06,39.92 B2.-
  Bottom 0.406: Q3.2 40.69,40.79 v40.69,38.65 40.7,38.64 40.7,38.32 R13.1 42.29,37.06 44.19,35.16 R12.1 44.5,34.84 43.23,33.57 37.51,33.57 36.88,34.21 C11.2 | Q1.2 59.36,44.11 59.99,43.48 59.99,37.32 C9.2 59.74,37.38 v58.47,38.65 57.51,39.61 U8.6
  Bottom 0.813: U1.B- 56.31,23.29 60.25,23.29 62.15,25.19 | 62.15,25.19 65.33,28.37 77.44,28.37 80.5,31.42 B2.- | 62.15,25.19 62.15,35.34 60.73,37.06 C9.2
  pour Bottom: 62.15,25.32 65.33,28.37 62.15,31.54
N$39
  Bottom 0.406: U4.5 U4.4 27.12,53.89 21.17,53.89 19.95,52.67 17.41,52.67 11.57,46.83 S5.P$3
  Bottom 0.61: C1.1 30.21,54.79 29.26,53.84 U4.5
  Bottom 0.813: L1.2 37.13,55.35 36.28,54.5 32.84,54.5 31.93,55.42 C1.1
N$40  (via drill 0.35)
  Top 0.406: S3.2 70.92,0.55 50.85,0.55 47.36,4.04 v47.36,8.17
  Bottom 0.406: v47.36,8.17 Q4.2 45.45,10.2 45.13,9.88 C14.1 45.13,11.66 44.85,11.95 D6.C 44.88,12.92 44.55,13.25 41.25,13.25 40.69,12.69 SJ11.1
  Bottom 0.61: S3.2 73.15,2.79 SJ8.2 73.15,6.23 J12.-
N$41
  Top 0.61: J8.IN+ 43.86,16.43 U1.IN+ 46.18,4.39 D1.C
  Bottom 0.406: F2.1 55.61,3.73 45.52,3.73 U1.IN+
  Bottom 0.813: D3.C 84.38,33.8 77.88,27.3 66.17,27.3 56.56,17.7 48.94,17.7 J8.IN+
N$42
  Top 0.406: R3.2 J10.1
N$43
  Bottom 0.406: Q4.1 49.52,10.46 55.23,10.46 R17.2
N$44
  Bottom 0.406: D6.A 41.36,11.76 D7.P$1 42.88,6.01 53.02,6.01 R18.1 R17.1 56.95,7.22 58.72,9 58.98,9 F2.2
N$45
  Top 0.61: D1.A 48.85,13.63 F1.1
N$46
  Bottom 0.406: U7.3 70.22,30.72 69.77,30.27 66.85,30.27 66.01,31.11 66.01,37.87 SJ9.1 65.86,37.94 64.44,39.36 SJ10.1
N$47  (via drill 0.35)
  Top 0.406: J19.SCLK 23.73,11.17 39.37,11.17 41.71,13.51 41.71,17.52 44.63,20.44 v44.63,21.51 | v51.48,22.14 61.64,22.14 v64.18,19.6
  Bottom 0.406: J11.SCLK 69.9,19.6 v64.18,19.6 | v44.63,21.51 45.26,22.14 v51.48,22.14
N$48  (via drill 0.35)
  Top 0.406: J19.MOSI 20.85,12.29 38.55,12.29 40.41,14.14 40.41,17.85 43.1,20.55 v43.1,20.75
  Bottom 0.406: J11.MOSI 69.9,22.14 62.38,22.14 56.66,16.43 47.42,16.43 v43.1,20.75
N$49
  Top 0.406: J19.CS 16,8.17 20.96,3.22 31.8,3.22 37.51,8.93 U3.2
  Bottom 0.406: U2.2 U3.2 | U2.2 56.82,14.78 58.47,16.43 65.45,16.43 J11.A2 | U2.2 39.42,18.62 J7.SIG 39.42,21.16 R15.1
N$50  (via drill 0.35)
  Top 0.406: J19.MISO 22.29,11.73 38.91,11.73 41.07,13.89 41.07,17.68 43.86,20.47 v43.86,22.78 | v64.18,23.41 v50.21,23.41
  Bottom 0.406: J11.MISO v64.18,23.41 | v43.86,22.78 44.5,23.41 v50.21,23.41
VCC  (via drill 0.35)
  Top 0.61: SJ3.1@V S4.10 | v80.69,24.68 79.42,24.68 78.15,25.95 78.15,30.4 v72.69,36.11
  other vias: 19.1,53.89
  pour Bottom (isolate 0.305, rank 5): -1.92,58.5 -1.92,-1.56 90.86,-1.56 90.86,58.5

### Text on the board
Bottom: v4.1
tPlace: AIN | GND | 10068-BCS-A4a v4.1 | MISO | MOSI | SDA | SCL | GND | Vcc | RX0 | SCLK | A0 | TX0 | In+ | In- | Bat- | Bat+ | SDA | A1 | Vcc | GND | SCL | SDA | RST | ADD | A2 | SCL | CSB / SDO / WAK | SDO / CS / INT | A3 | Vcc | D+ | D-
bPlace: Rx | Vin+ | Vin- | SDA | SCL | GND | Vcc | digitalconcepts.net.au | GND | Tx | Vcc | S/N | 1 | 2 | 3 | 4
tNames: Timer Trim | J12 | ON
bNames: Vcc | GND | Boost | Bypass | Boost | J1 | J2
tValues: SDA | SCL | GND | Vcc | GND | Speed | Dir'n | Rain | Vcc | Monitor Bypass | TP5000 Interface | External / Power / Switch
bValues: MIC5219 / AP2112 | SDA | SCL | GND | Vcc | MOSFET / Bypass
